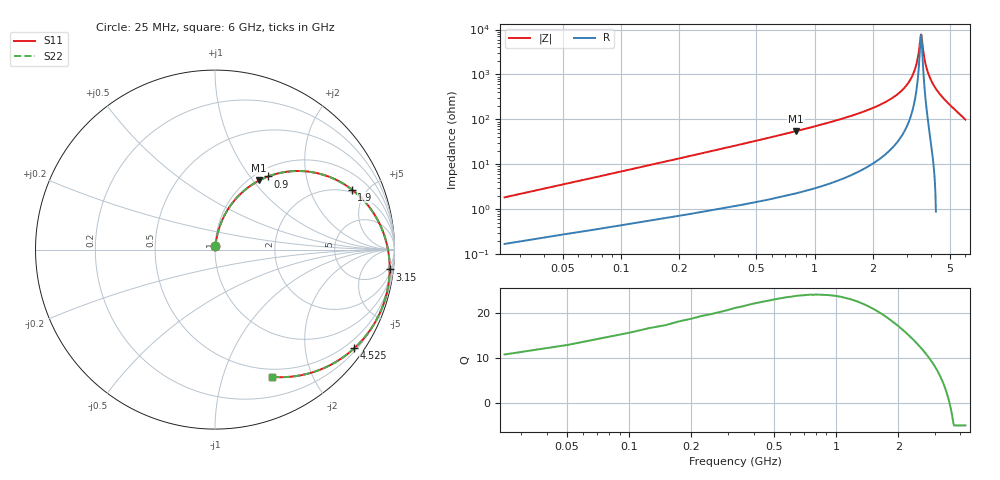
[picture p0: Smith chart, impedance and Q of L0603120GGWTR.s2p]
!	AVX Thin Film Operation
!	Date:	March	2003
!	Description: Accu-L® Series Thin Film SMD RF Inductors
!	Part Number: L0603120GGWTR
!	25MHz-6GHz
!	Serial	Measurements
#	mhz	S	db	R	50
!	S11	S11	S21	S21	S12	S12	S22	S22
!	dB	Phase	dB	Phase	dB	Phase	dB	Phase
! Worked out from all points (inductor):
!   240 points, 25 MHz to 6 GHz, reference 50 ohm
!   read as one part in series: L = 11.2 nH near 50 MHz
!   highest Q = 24.2 at 800 MHz (marker M1), where L = 10.9 nH
!   self-resonance near 3.525 GHz
!   S11 on the Smith chart (normalised r, x): 25 MHz: 1.00, +0.04; 900 MHz: 1.13, +1.23; 1.9 GHz: 1.82, +3.97; 3.15 GHz: 3, -17; 4.525 GHz: 0.27, -3.12; 6 GHz: 0.41, -1.46
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25  -35.02 83.3  -0.02 -1.1  -0.02 -1.1  -35.02 83.3
50  -29.33 83.3  -0.03 -2.1  -0.03 -2.1  -29.33 83.3
100  -23.59 82.0  -0.06 -4.1  -0.06 -4.1  -23.59 82.0
225  -16.87 77.8  -0.16 -9.0  -0.16 -9.0  -16.87 77.8
450  -11.22 69.7  -0.45 -17.5  -0.45 -17.5  -11.22 69.7
800  -6.79 57.4  -1.19 -30.0  -1.19 -30.0  -6.79 57.4
900  -5.95 54.0  -1.46 -33.3  -1.46 -33.3  -5.95 54.0
1025  -5.06 49.8  -1.84 -37.5  -1.84 -37.5  -5.06 49.8
1900  -1.59 23.7  -5.63 -62.8  -5.63 -62.8  -1.59 23.7
2025  -1.33 20.4  -6.36 -66.0  -6.36 -66.0  -1.33 20.4
2600  -0.53 6.1  -10.75 -79.1  -10.75 -79.1  -0.53 6.1
3025  -0.23 -3.7  -16.15 -86.4  -16.15 -86.4  -0.23 -3.7
3150  -0.18 -6.5  -18.59 -87.6  -18.59 -87.6  -0.18 -6.5
3375  -0.12 -11.4  -25.86 -84.4  -25.86 -84.4  -0.12 -11.4
3525  -0.11 -14.6  -37.41 -35.0  -37.41 -35.0  -0.11 -14.6
3550  -0.11 -15.1  -38.06 -3.3  -38.06 -3.3  -0.11 -15.1
3650  -0.11 -17.2  -29.60 54.1  -29.60 54.1  -0.11 -17.2
3725  -0.12 -18.8  -25.42 61.1  -25.42 61.1  -0.12 -18.8
4025  -0.19 -25.0  -17.31 63.3  -17.31 63.3  -0.19 -25.0
4525  -0.44 -35.3  -11.41 56.2  -11.41 56.2  -0.44 -35.3
5025  -0.85 -45.5  -8.12 47.6  -8.12 47.6  -0.85 -45.5
6000  -2.20 -66.0  -4.32 29.9  -4.32 29.9  -2.20 -66.0
